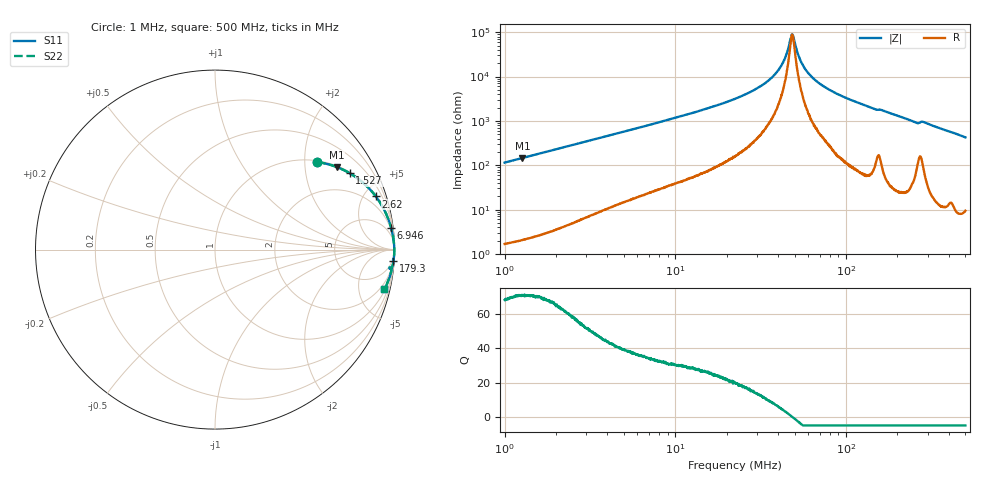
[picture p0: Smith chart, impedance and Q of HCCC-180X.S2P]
!s-Parameter Generated by FASTRON Sdn. Bhd.
!FASTRON P/N : HCCC-180X
!Keysight Technologies,E4991B,MY54100416,A.01.15
!Date: Mon Apr 06 15:53:25 2026
!Version  : Rev00 Mon Apr 06 15:53:25 2026
!Data & Calibration Information:
!PortZ  Port1:50+j0  Port2:50+j0
!When reading, reference impedance value at option line is always used.
! Remarks : This data is being provided solely for informational purposes.
!Freq	S11	S21	S12	S22
# Hz S dB R 50
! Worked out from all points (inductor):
!   1601 points, 1 MHz to 500 MHz, reference 50 ohm
!   read as one part in series: L = 18.3 uH near 1.032 MHz
!   highest Q = 70.8 at 1.272 MHz (marker M1), where L = 18.3 uH
!   self-resonance near 48.25 MHz
!   S11 on the Smith chart (normalised r, x): 1 MHz: 1.03, +2.30; 1.527 MHz: 1.05, +3.50; 2.62 MHz: 1.11, +6.02; 6.946 MHz: 1, +16; 179.3 MHz: 2, -30; 500 MHz: 1.19, -8.51
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1000000  -2.52 40.7  -3.71 -48.5  -3.71 -48.5  -2.52 40.7
1272287  -1.73 34.1  -5.02 -55.0  -5.02 -55.0  -1.73 34.1
1527099  -1.28 29.5  -6.15 -59.7  -6.15 -59.7  -1.28 29.5
2620236  -0.50 18.3  -10.07 -70.7  -10.07 -70.7  -0.50 18.3
2820919  -0.44 17.1  -10.65 -71.9  -10.65 -71.9  -0.44 17.1
6946104  -0.10 7.1  -18.17 -81.2  -18.17 -81.2  -0.10 7.1
7957584  -0.08 6.2  -19.38 -82.1  -19.38 -82.1  -0.08 6.2
2.236068e7  -0.02 1.8  -29.98 -85.3  -29.98 -85.3  -0.02 1.8
3.074732e7  -0.01 1.0  -35.13 -84.5  -35.13 -84.5  -0.01 1.0
3.792254e7  -0.01 0.5  -40.65 -82.0  -40.65 -82.0  -0.01 0.5
4.294146e7  -0.01 0.3  -46.76 -75.3  -46.76 -75.3  -0.01 0.3
4.481592e7  -0.01 0.2  -50.21 -68.6  -50.21 -68.6  -0.01 0.2
4.732038e7  -0.01 0.0  -57.02 -37.1  -57.02 -37.1  -0.01 0.0
4.824836e7  -0.01 0.0  -59.01 -4.2  -59.01 -4.2  -0.01 0.0
4.938598e7  -0.01 -0.0  -57.39 34.3  -57.39 34.3  -0.01 -0.0
5.25525e7  -0.01 -0.2  -49.71 70.0  -49.71 70.0  -0.01 -0.2
5.505993e7  -0.01 -0.3  -46.05 77.0  -46.05 77.0  -0.01 -0.3
6.307767e7  -0.01 -0.6  -39.80 83.5  -39.80 83.5  -0.01 -0.6
9.193919e7  -0.01 -1.5  -31.64 86.3  -31.64 86.3  -0.01 -1.5
1.77937e8  -0.03 -3.7  -23.74 84.9  -23.74 84.9  -0.03 -3.7
1.793246e8  -0.03 -3.8  -23.65 84.9  -23.65 84.9  -0.03 -3.8
5e8  -0.28 -13.1  -12.86 75.6  -12.86 75.6  -0.28 -13.1
